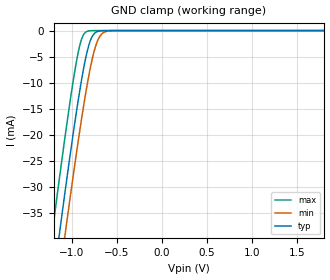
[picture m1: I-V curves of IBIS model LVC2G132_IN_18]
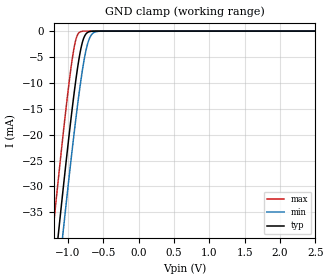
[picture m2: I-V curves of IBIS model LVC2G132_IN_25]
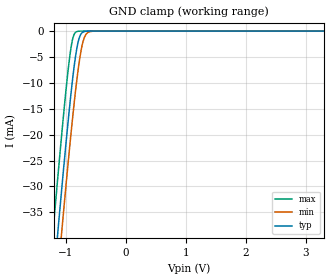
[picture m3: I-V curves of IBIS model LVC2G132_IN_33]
| TEXAS INSTRUMENTS INCORPORATED
| Standard Linear and Logic Group
| IBIS Model of SN74LVC2G132
| Dual 2-Input NAND gate with Schmitt-trigger Inputs
| This file contains package information for the following:
|  SOT 8-pin (DCT) package as [Component] LVC2G132_DCT
|  SOT 8-pin (DCU) package as [Component] LVC2G132_DCU
|  NanoStar WCSP 8-pin (YEP) package as [Component] LVC2G132_YEP
|  NanoFree WCSP 8-pin (YZP) package as [Component] LVC2G132_YZP
| This device can be powered at the following Vccs:
|  1.8 volt Vcc
|  2.5 volt Vcc
|  3.3 volt Vcc
|  5 volt Vcc
| This file provides unique models under the [Model Selector] for each Vcc.
| For operation at a specific Vcc, select the appropriate model after each
| [Model Selector] keyword.
[IBIS Ver]   3.2
[Comment char]  |_char
[File Name]   sn74lvc2g132.ibs
[File Rev]   1.2 | x_die
[Date]   12/11/2003
[Source]   Data created from TI-SPICE simulations at TI-SLL.
[Notes]   The following is an IBIS list for the LVC2G132.
   Please contact sllibis@ti.com with questions and
   comments concerning SLL IBIS models
   - FILE REV HISTORY
   - 1.1 Release IBIS file on 12/11/03
   - 1.2 YEP and YZP packages released on 10/27/04
   - Non-monotonic data in pullup, pulldown due to
   over-voltage-tolerant circuit.
   - Power clamp data deleted as there is no power-clamp diode.
[Disclaimer] Property of Texas Instruments Incorporated.  Unauthorized
   reproduction and/or distribution is strictly prohibited.
   This product is protected under copyright law.
   Created  2003, (C) Copyright  2003, Texas Instruments
   Incorporated, All Rights Reserved
   UNLESS THERE IS A SIGNED, WRITTEN AGREEMENT TO THE
   CONTRARY, TEXAS INSTRUMENTS (TI) IS PROVIDING THE IBIS
   MODELS  AND WITHOUT ANY WARRANTY, EXPRESSED OR
   IMPLIED.  TI assumes no liability for:
   1) the accuracy of the IBIS models provided to your
   company;
   2) the proper functioning of these IBIS Models in your
   design or for any resulting applications; or
   3) infringement of patents, copyrights or intellectual
   property rights resulting from your use of these IBIS
   models.
   TI provides IBIS Models as a service to our customers.
   You and your company shall not distribute, sell or give
   these models to anyone else without prior written
   permission from TI.
   TI reserves the right to make changes to our products or
   to discontinue any semiconductor product or service
   without notice, and advises our customers to obtain the
   latest version of relevant information to verify, before
   placing orders, that the information being relied on is
   current.
   Please be aware that your receipt and use of the IBIS
   information provided shall serve as acceptance of these
   terms and conditions.  If you do not accept these terms,
   you should return or destroy the IBIS models and any
   other accompanying information immediately.
| Component LVC2G132_DCT 8-pin SOT
[Component]   LVC2G132_DCT
[Manufacturer]   Texas Instruments, Inc.
[Package]
|   typ   min   max
R_pkg   2.900e-02   2.800e-02   3.100e-02
L_pkg   1.796e-09   1.666e-09   1.924e-09
C_pkg   2.310e-13   2.210e-13   2.420e-13
[Pin]   signal_name   model_name   R_pin   L_pin   C_pin
1   1A   LVC2G132_IN   3.100e-02   1.894e-09   2.230e-13
2   1B   LVC2G132_IN   2.800e-02   1.697e-09   2.370e-13
3   2Y   LVC2G132_OUT   3.000e-02   1.722e-09   2.390e-13
4   GND   GND   3.000e-02   1.861e-09   2.210e-13
5   2A   LVC2G132_IN   2.800e-02   1.924e-09   2.280e-13
6   2B   LVC2G132_IN   2.900e-02   1.736e-09   2.420e-13
7   1Y   LVC2G132_OUT   2.800e-02   1.666e-09   2.360e-13
8   VCC   POWER   3.000e-02   1.871e-09   2.220e-13
| Component LVC2G132_DCU 8-pin SOT
[Component]   LVC2G132_DCU
[Manufacturer]   Texas Instruments, Inc.
[Package]
|   typ   min   max
R_pkg   2.600e-02   2.300e-02   3.800e-02
L_pkg   1.394e-09   1.066e-09   2.046e-09
C_pkg   2.590e-13   2.150e-13   3.720e-13
[Pin]   signal_name   model_name   R_pin   L_pin   C_pin
1   1A   LVC2G132_IN   2.400e-02   1.520e-09   2.710e-13
2   1B   LVC2G132_IN   2.300e-02   1.112e-09   2.180e-13
3   2Y   LVC2G132_OUT   2.300e-02   1.070e-09   2.170e-13
4   GND   GND   2.700e-02   2.046e-09   3.720e-13
5   2A   LVC2G132_IN   2.700e-02   1.542e-09   2.730e-13
6   2B   LVC2G132_IN   2.300e-02   1.100e-09   2.240e-13
7   1Y   LVC2G132_OUT   2.300e-02   1.066e-09   2.150e-13
8   VCC   POWER   3.800e-02   1.696e-09   2.800e-13
| Component LVC2G132_YEP 8-pin NanoStar WCSP
[Component]   LVC2G132_YEP
[Manufacturer]   Texas Instruments, Inc.
[Package]
|   typ   min   max
R_pkg   0.001   0.001   0.001
L_pkg   0.021nH   0.021nH   0.021nH
C_pkg   0.043pF   0.042pF   0.044pF
[Pin]   signal_name   model_name   R_pin   L_pin   C_pin
1   1A   LVC2G132_IN   0.046   2.861nH   0.321pF
2   1B   LVC2G132_IN   0.037   2.437nH   0.286pF
3   2Y   LVC2G132_OUT   0.034   2.419nH   0.286pF
4   GND   GND   0.043   2.784nH   0.321pF
5   2A   LVC2G132_IN   0.043   2.784nH   0.321pF
6   2B   LVC2G132_IN   0.035   2.420nH   0.286pF
7   1Y   LVC2G132_OUT   0.037   2.437nH   0.286pF
8   VCC   POWER   0.046   2.860nH   0.321pF
| Component LVC2G132_YZP 8-pin NanoFree WCSP
[Component]   LVC2G132_YZP
[Manufacturer]   Texas Instruments, Inc.
[Package]
|   typ   min   max
R_pkg   0.001   0.001   0.001
L_pkg   0.021nH   0.021nH   0.021nH
C_pkg   0.043pF   0.042pF   0.044pF
[Pin]   signal_name   model_name   R_pin   L_pin   C_pin
1   1A   LVC2G132_IN   0.046   2.861nH   0.321pF
2   1B   LVC2G132_IN   0.037   2.437nH   0.286pF
3   2Y   LVC2G132_OUT   0.034   2.419nH   0.286pF
4   GND   GND   0.043   2.784nH   0.321pF
5   2A   LVC2G132_IN   0.043   2.784nH   0.321pF
6   2B   LVC2G132_IN   0.035   2.420nH   0.286pF
7   1Y   LVC2G132_OUT   0.037   2.437nH   0.286pF
8   VCC   POWER   0.046   2.860nH   0.321pF
| Model LVC2G132_IN
[Model Selector]   LVC2G132_IN
LVC2G132_IN_18   1.8 volt Vcc
LVC2G132_IN_25   2.5 volt Vcc
LVC2G132_IN_33   3.3 volt Vcc
LVC2G132_IN_50   5 volt Vcc
| Model LVC2G132_OUT
[Model Selector]   LVC2G132_OUT
LVC2G132_OUT_18   1.8 volt Vcc
LVC2G132_OUT_25   2.5 volt Vcc
LVC2G132_OUT_33   3.3 volt Vcc
LVC2G132_OUT_50   5 volt Vcc
| Models and submodels in the file (8): LVC2G132_IN_18 (Input), LVC2G132_IN_25 (Input), LVC2G132_IN_33 (Input), LVC2G132_IN_50 (Input), LVC2G132_OUT_18 (Output), LVC2G132_OUT_25 (Output), LVC2G132_OUT_33 (Output), LVC2G132_OUT_50 (Output)
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[Model]   LVC2G132_IN_18
Model_type  Input
Vinl=0.5775
Vinh=1.2675
| variable   typ   min   max
C_comp   3.55pF   2.93pF   4.36pF
[Temperature Range]   40   100   -40
| Ambient temperature   25   85   -40
[Voltage range]   1.8   1.65   1.95
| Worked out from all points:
|   GND clamp passes 1 mA (typ) near -0.77 V on its own axis
[GND Clamp]
| LVC2G132_IN_18
|   Voltage   I(typ)   I(min)   I(max)
-5.5V     -655.2mA   -662.2mA   -646.6mA
-1.215V   -49.6mA    -57.88mA   -38.96mA
-1.135V   -39.07mA   -47.36mA   -28.42mA
-1.075V   -31.35mA   -39.6mA    -20.75mA
-1.055V   -28.82mA   -37.05mA   -18.27mA
-955mV    -16.68mA   -24.66mA   -6.874mA
-885mV    -9.098mA   -16.55mA   -1.486mA
-825mV    -3.922mA   -10.26mA   -137.1uA
-780mV    -1.472mA   -6.227mA   -17.15uA
-715mV    -205.4uA   -2.128mA   -808.5nA
-650mV    -22.01uA   -443.9uA   -37.93nA
1.8V      3.326pA    6.142pA    3.026pA
[Model]   LVC2G132_IN_25
Model_type  Input
Vinl=0.7
Vinh=1.7
| variable   typ   min   max
C_comp   3.52pF   3.00pF   4.41pF
[Temperature Range]   40   100   -40
| Ambient temperature   25   85   -40
[Voltage range]   2.5   2.3   2.7
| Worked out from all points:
|   GND clamp passes 1 mA (typ) near -0.77 V on its own axis
[GND Clamp]
| LVC2G132_IN_25
|   Voltage   I(typ)   I(min)   I(max)
-5.5V     -655.2mA   -662.2mA   -646.6mA
-1.215V   -49.6mA    -57.88mA   -38.96mA
-1.14V    -39.72mA   -48.01mA   -29.07mA
-1.12V    -37.12mA   -45.41mA   -26.48mA
-1.08V    -31.98mA   -40.25mA   -21.38mA
-1.06V    -29.44mA   -37.69mA   -18.89mA
-960mV    -17.26mA   -25.26mA   -7.377mA
-890mV    -9.597mA   -17.1mA    -1.734mA
-785mV    -1.671mA   -6.635mA   -21.67uA
-720mV    -242.5uA   -2.354mA   -1.023uA
-650mV    -22.01uA   -443.9uA   -37.93nA
2.5V      4.713pA    7.577pA    4.389pA
[Model]   LVC2G132_IN_33
Model_type  Input
Vinl=0.8
Vinh=2.0
| variable   typ   min   max
C_comp   3.46pF   2.86pF   4.52pF
[Temperature Range]   40   100   -40
| Ambient temperature   25   85   -40
[Voltage range]   3.3   3   3.6
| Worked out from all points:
|   GND clamp passes 1 mA (typ) near -0.77 V on its own axis
[GND Clamp]
| LVC2G132_IN_33
|   Voltage   I(typ)   I(min)   I(max)
-5.5V     -655.2mA   -662.2mA   -646.6mA
-1.225V   -50.93mA   -59.21mA   -40.3mA
-1.145V   -40.37mA   -48.66mA   -29.72mA
-1.12V    -37.12mA   -45.41mA   -26.48mA
-1.08V    -31.98mA   -40.25mA   -21.38mA
-1.06V    -29.44mA   -37.69mA   -18.89mA
-965mV    -17.84mA   -25.87mA   -7.89mA
-885mV    -9.098mA   -16.55mA   -1.486mA
-780mV    -1.472mA   -6.227mA   -17.15uA
-715mV    -205.4uA   -2.128mA   -808.5nA
-640mV    -15.53uA   -338.1uA   -23.69nA
3.3V      6.304pA    9.258pA    5.93pA
